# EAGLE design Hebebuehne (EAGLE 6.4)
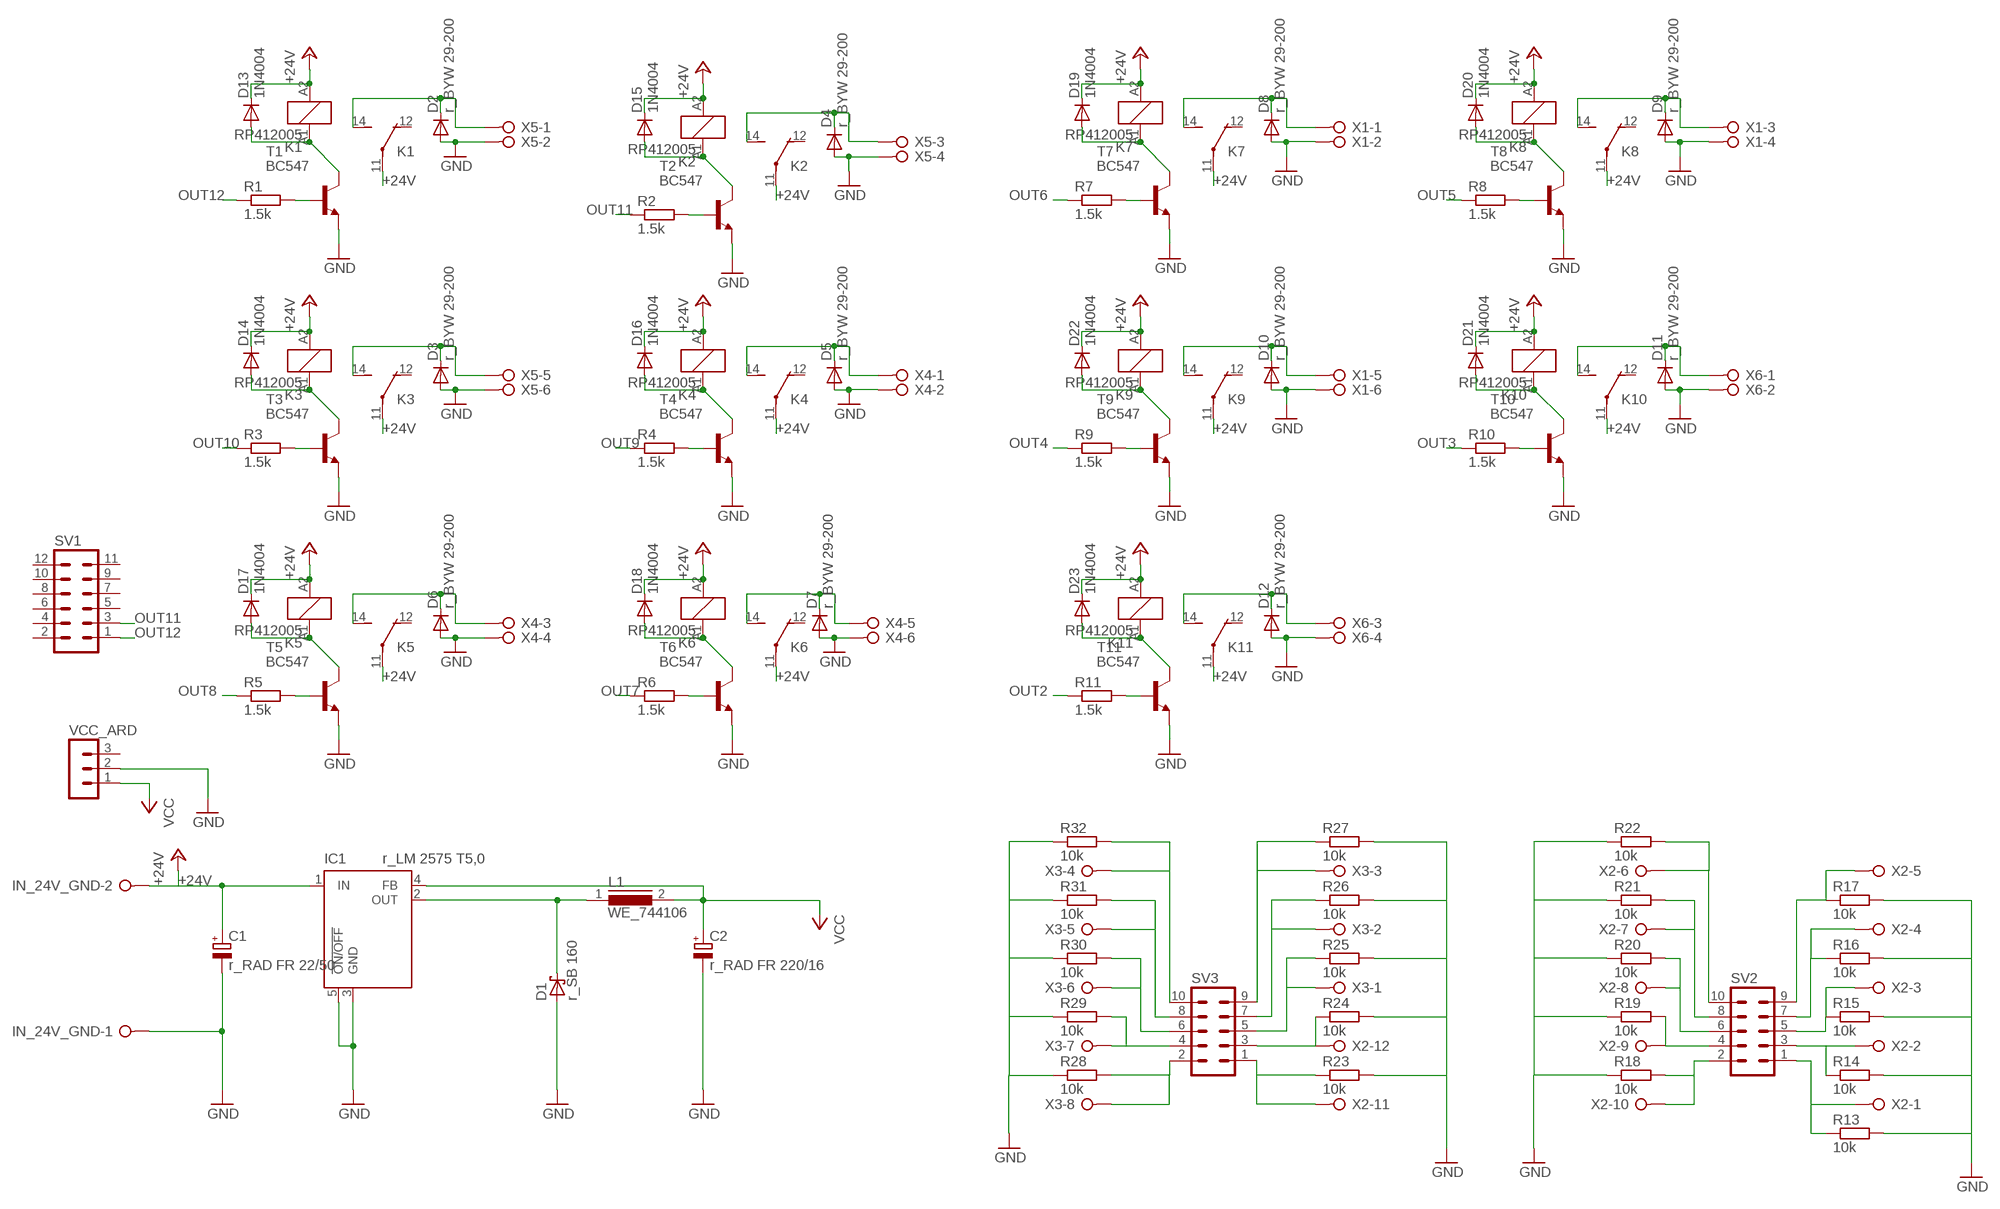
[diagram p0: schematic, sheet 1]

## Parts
C1  r_RAD FR 22/50  CPOL-EUE2.5-6  [E2,5-6]
C2  r_RAD FR 220/16  CPOL-EUE2.5-6  [E2,5-6]
D1  r_SB 160  BAT49  [DO41-10]
D2  r_BYW 29-200  MUR810  [TO220ACS]
D3  r_BYW 29-200  MUR810  [TO220ACS]
D4  r_BYW 29-200  MUR810  [TO220ACS]
D5  r_BYW 29-200  MUR810  [TO220ACS]
D6  r_BYW 29-200  MUR810  [TO220ACS]
D7  r_BYW 29-200  MUR810  [TO220ACS]
D8  r_BYW 29-200  MUR810  [TO220ACS]
D9  r_BYW 29-200  MUR810  [TO220ACS]
D10  r_BYW 29-200  MUR810  [TO220ACS]
D11  r_BYW 29-200  MUR810  [TO220ACS]
D12  r_BYW 29-200  MUR810  [TO220ACS]
D13  1N4004  [DO41-10]
D14  1N4004  [DO41-10]
D15  1N4004  [DO41-10]
D16  1N4004  [DO41-10]
D17  1N4004  [DO41-10]
D18  1N4004  [DO41-10]
D19  1N4004  [DO41-10]
D20  1N4004  [DO41-10]
D21  1N4004  [DO41-10]
D22  1N4004  [DO41-10]
D23  1N4004  [DO41-10]
IC1  r_LM 2575 T5,0  LM2575  [CB367]
IN_24V_GND  W237-02P  [W237-132]
K1  RP412005  [RT-C/O12A3.5]
K2  RP412005  [RT-C/O12A3.5]
K3  RP412005  [RT-C/O12A3.5]
K4  RP412005  [RT-C/O12A3.5]
K5  RP412005  [RT-C/O12A3.5]
K6  RP412005  [RT-C/O12A3.5]
K7  RP412005  [RT-C/O12A3.5]
K8  RP412005  [RT-C/O12A3.5]
K9  RP412005  [RT-C/O12A3.5]
K10  RP412005  [RT-C/O12A3.5]
K11  RP412005  [RT-C/O12A3.5]
L1  WE_744106  R1305D11  [11-13]
R1  1.5k  R-EU_0204/7  [0204/7]
R2  1.5k  R-EU_0204/7  [0204/7]
R3  1.5k  R-EU_0204/7  [0204/7]
R4  1.5k  R-EU_0204/7  [0204/7]
R5  1.5k  R-EU_0204/7  [0204/7]
R6  1.5k  R-EU_0204/7  [0204/7]
R7  1.5k  R-EU_0204/7  [0204/7]
R8  1.5k  R-EU_0204/7  [0204/7]
R9  1.5k  R-EU_0204/7  [0204/7]
R10  1.5k  R-EU_0204/7  [0204/7]
R11  1.5k  R-EU_0204/7  [0204/7]
R13  10k  R-EU_0207/10  [0207/10]
R14  10k  R-EU_0207/10  [0207/10]
R15  10k  R-EU_0207/10  [0207/10]
R16  10k  R-EU_0207/10  [0207/10]
R17  10k  R-EU_0207/10  [0207/10]
R18  10k  R-EU_0207/10  [0207/10]
R19  10k  R-EU_0207/10  [0207/10]
R20  10k  R-EU_0207/10  [0207/10]
R21  10k  R-EU_0207/10  [0207/10]
R22  10k  R-EU_0207/10  [0207/10]
R23  10k  R-EU_0207/10  [0207/10]
R24  10k  R-EU_0207/10  [0207/10]
R25  10k  R-EU_0207/10  [0207/10]
R26  10k  R-EU_0207/10  [0207/10]
R27  10k  R-EU_0207/10  [0207/10]
R28  10k  R-EU_0207/10  [0207/10]
R29  10k  R-EU_0207/10  [0207/10]
R30  10k  R-EU_0207/10  [0207/10]
R31  10k  R-EU_0207/10  [0207/10]
R32  10k  R-EU_0207/10  [0207/10]
SV1  MA06-2  [MA06-2]
SV2  MA05-2  [MA05-2]
SV3  MA05-2  [MA05-2]
T1  BC547  [TO92]
T2  BC547  [TO92]
T3  BC547  [TO92]
T4  BC547  [TO92]
T5  BC547  [TO92]
T6  BC547  [TO92]
T7  BC547  [TO92]
T8  BC547  [TO92]
T9  BC547  [TO92]
T10  BC547  [TO92]
T11  BC547  [TO92]
VCC_ARD  MA03-1  [MA03-1]
X1  W237-06P  [W237-6P]
X2  W237-12P  [W237-12P]
X3  W237-08P  [W237-8P]
X4  W237-06P  [W237-6P]
X5  W237-06P  [W237-6P]
X6  W237-04P  [W237-4P]

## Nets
+24V: C1.+ D13.C D14.C D15.C D16.C D17.C D18.C D19.C D20.C D21.C D22.C D23.C IC1.1(IN) IN_24V_GND.2 K1.11(2:P) K1.A2 K2.11(2:P) K2.A2 K3.11(2:P) K3.A2 K4.11(2:P) K4.A2 K5.11(2:P) K5.A2 K6.11(2:P) K6.A2 K7.11(2:P) K7.A2 K8.11(2:P) K8.A2 K9.11(2:P) K9.A2 K10.11(2:P) K10.A2 K11.11(2:P) K11.A2
GND: C1.- C2.- D1.A D2.A D3.A D4.A D5.A D6.A D7.A D8.A D9.A D10.A D11.A D12.A IC1.3(GND) IC1.5(!ON/OFF) IN_24V_GND.1 R13.2 R14.2 R15.2 R16.2 R17.2 R18.1 R19.1 R20.1 R21.1 R22.1 R23.2 R24.2 R25.2 R26.2 R27.2 R28.1 R29.1 R30.1 R31.1 R32.1 T1.1(E) T2.1(E) T3.1(E) T4.1(E) T5.1(E) T6.1(E) T7.1(E) T8.1(E) T9.1(E) T10.1(E) T11.1(E) VCC_ARD.2 X1.2 X1.4 X1.6 X4.2 X4.4 X4.6 X5.2 X5.4 X5.6 X6.2 X6.4
N$1: D5.C K4.14(2:S) X4.1
N$2: D2.C K1.14(2:S) X5.1
N$3: D1.C IC1.2(OUT) L1.1
N$4: D4.C K2.14(2:S) X5.3
N$5: D3.C K3.14(2:S) X5.5
N$6: R1.2 T1.2(B)
N$7: D13.A K1.A1 T1.3(C)
N$8: R2.2 T2.2(B)
N$9: D6.C K5.14(2:S) X4.3
N$10: D7.C K6.14(2:S) X4.5
N$11: D8.C K7.14(2:S) X1.1
N$12: D15.A K2.A1 T2.3(C)
N$13: R3.2 T3.2(B)
N$14: R9.2 T9.2(B)
N$15: D9.C K8.14(2:S) X1.3
N$16: D22.A K9.A1 T9.3(C)
N$17: D14.A K3.A1 T3.3(C)
N$18: R4.2 T4.2(B)
N$19: R10.2 T10.2(B)
N$20: D21.A K10.A1 T10.3(C)
N$21: D10.C K9.14(2:S) X1.5
N$22: D16.A K4.A1 T4.3(C)
N$23: R5.2 T5.2(B)
N$24: D11.C K10.14(2:S) X6.1
N$25: R11.2 T11.2(B)
N$26: D23.A K11.A1 T11.3(C)
N$27: D17.A K5.A1 T5.3(C)
N$28: R6.2 T6.2(B)
N$31: D12.C K11.14(2:S) X6.3
N$32: D18.A K6.A1 T6.3(C)
N$33: R7.2 T7.2(B)
N$35: R28.2 SV3.2 X3.8
N$36: R29.2 SV3.4 X3.7
N$37: D19.A K7.A1 T7.3(C)
N$38: R8.2 T8.2(B)
N$39: R22.2 SV2.10 X2.6
N$40: R32.2 SV3.10 X3.4
N$41: R31.2 SV3.8 X3.5
N$42: D20.A K8.A1 T8.3(C)
N$43: R21.2 SV2.8 X2.7
N$44: R20.2 SV2.6 X2.8
N$45: R15.1 SV2.5 X2.3
N$46: R17.1 SV2.9 X2.5
N$47: R16.1 SV2.7 X2.4
N$48: R14.1 SV2.3 X2.2
N$49: R13.1 SV2.1 X2.1
N$50: R30.2 SV3.6 X3.6
N$51: R19.2 SV2.4 X2.9
N$52: R18.2 SV2.2 X2.10
N$53: R23.1 SV3.1 X2.11
N$54: R24.1 SV3.3 X2.12
N$55: R27.1 SV3.9 X3.3
N$56: R26.1 SV3.7 X3.2
N$57: R25.1 SV3.5 X3.1
OUT2: R11.1
OUT3: R10.1
OUT4: R9.1
OUT5: R8.1
OUT6: R7.1
OUT7: R6.1
OUT8: R5.1
OUT9: R4.1
OUT10: R3.1
OUT11: R2.1 SV1.3
OUT12: R1.1 SV1.1
VCC: C2.+ IC1.4(FB) L1.2 VCC_ARD.1
Unconnected: K1.12(2:O) K2.12(2:O) K3.12(2:O) K4.12(2:O) K5.12(2:O) K6.12(2:O) K7.12(2:O) K8.12(2:O) K9.12(2:O) K10.12(2:O) K11.12(2:O) SV1.2 SV1.4 SV1.5 SV1.6 SV1.7 SV1.8 SV1.9 SV1.10 SV1.11 SV1.12 VCC_ARD.3

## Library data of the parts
C1 C2 = resistor:CPOL-EU: POLARIZED CAPACITOR, European symbol
D1 = diode:BAT49: DIODE
D2-D12 = diode:MUR810: DIODE
D13-D23 = diode:1N4004: DIODE
IC1 = eigene:LM2575
IN_24V_GND = con-wago-508:W237-02P: WAGO SREW CLAMP; OC_FARNELL: unknown; OC_NEWARK: unknown
K1-K11 = relay:RP?12*: Power PCB Relay RP II/1 SCHRACK 1 pole 8 / 12 A Source: http://www.schrack.com/.. 5834.pdf; MF: TYCO ELECTRONICS; MPN: 1393231-8; OC_FARNELL: unknown; OC_NEWARK: 11H3247
L1 = inductor-nkl:R1305D: Speicherdrossel (bis typ. 250kHz); OC_FARNELL: unknown; OC_NEWARK: unknown
R1-R11 R13-R32 = resistor:R-EU_: RESISTOR, European symbol
SV1 = con-lstb:MA06-2: PIN HEADER; OC_FARNELL: unknown; OC_NEWARK: unknown
SV2 SV3 = con-lstb:MA05-2: PIN HEADER; OC_FARNELL: unknown; OC_NEWARK: unknown
T1-T11 = transistor:BC547: NPN TRANSISTOR
VCC_ARD = con-lstb:MA03-1: PIN HEADER; OC_FARNELL: unknown; OC_NEWARK: unknown
X1 X4 X5 = con-wago-508:W237-06P: WAGO SREW CLAMP; OC_FARNELL: unknown; OC_NEWARK: unknown
X2 = con-wago-508:W237-12P: WAGO SREW CLAMP; OC_FARNELL: unknown; OC_NEWARK: unknown
X3 = con-wago-508:W237-08P: WAGO SREW CLAMP; OC_FARNELL: unknown; OC_NEWARK: unknown
X6 = con-wago-508:W237-04P: WAGO SREW CLAMP; OC_FARNELL: unknown; OC_NEWARK: unknown

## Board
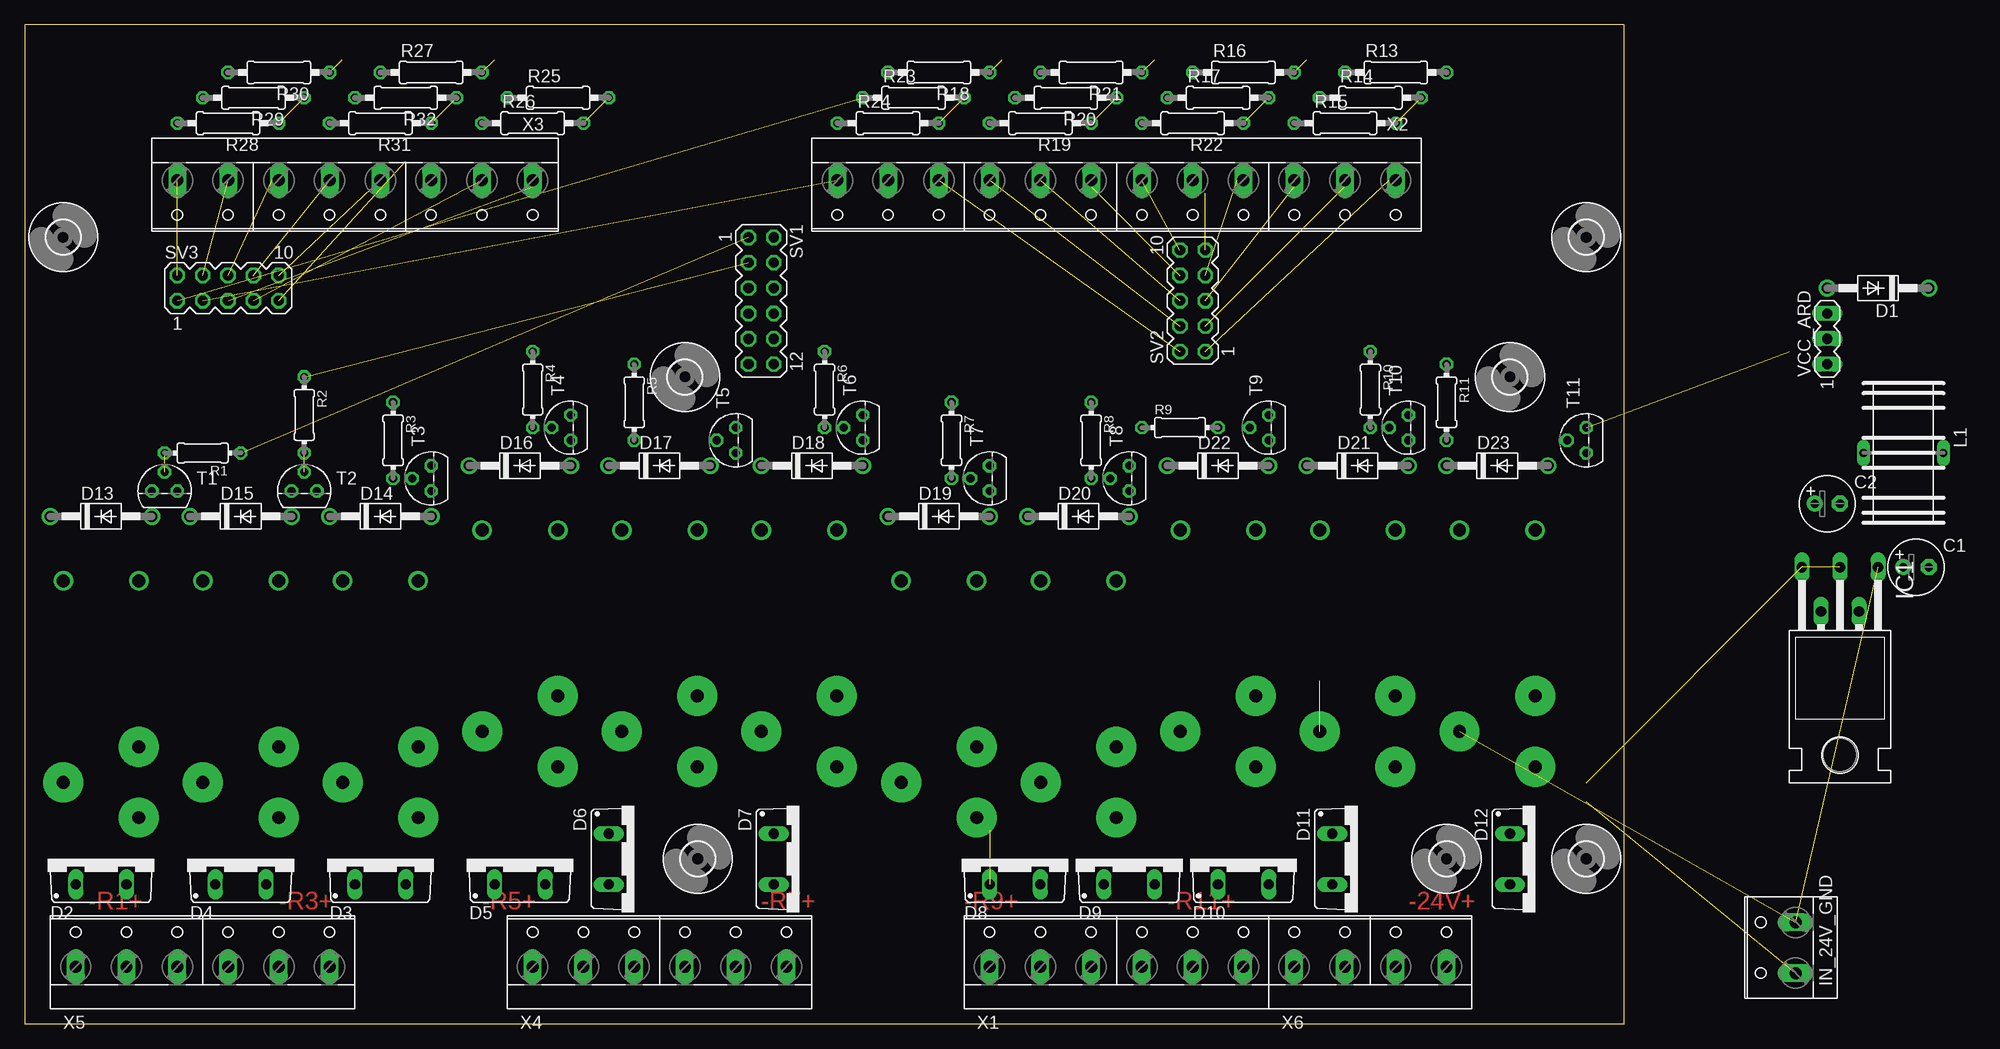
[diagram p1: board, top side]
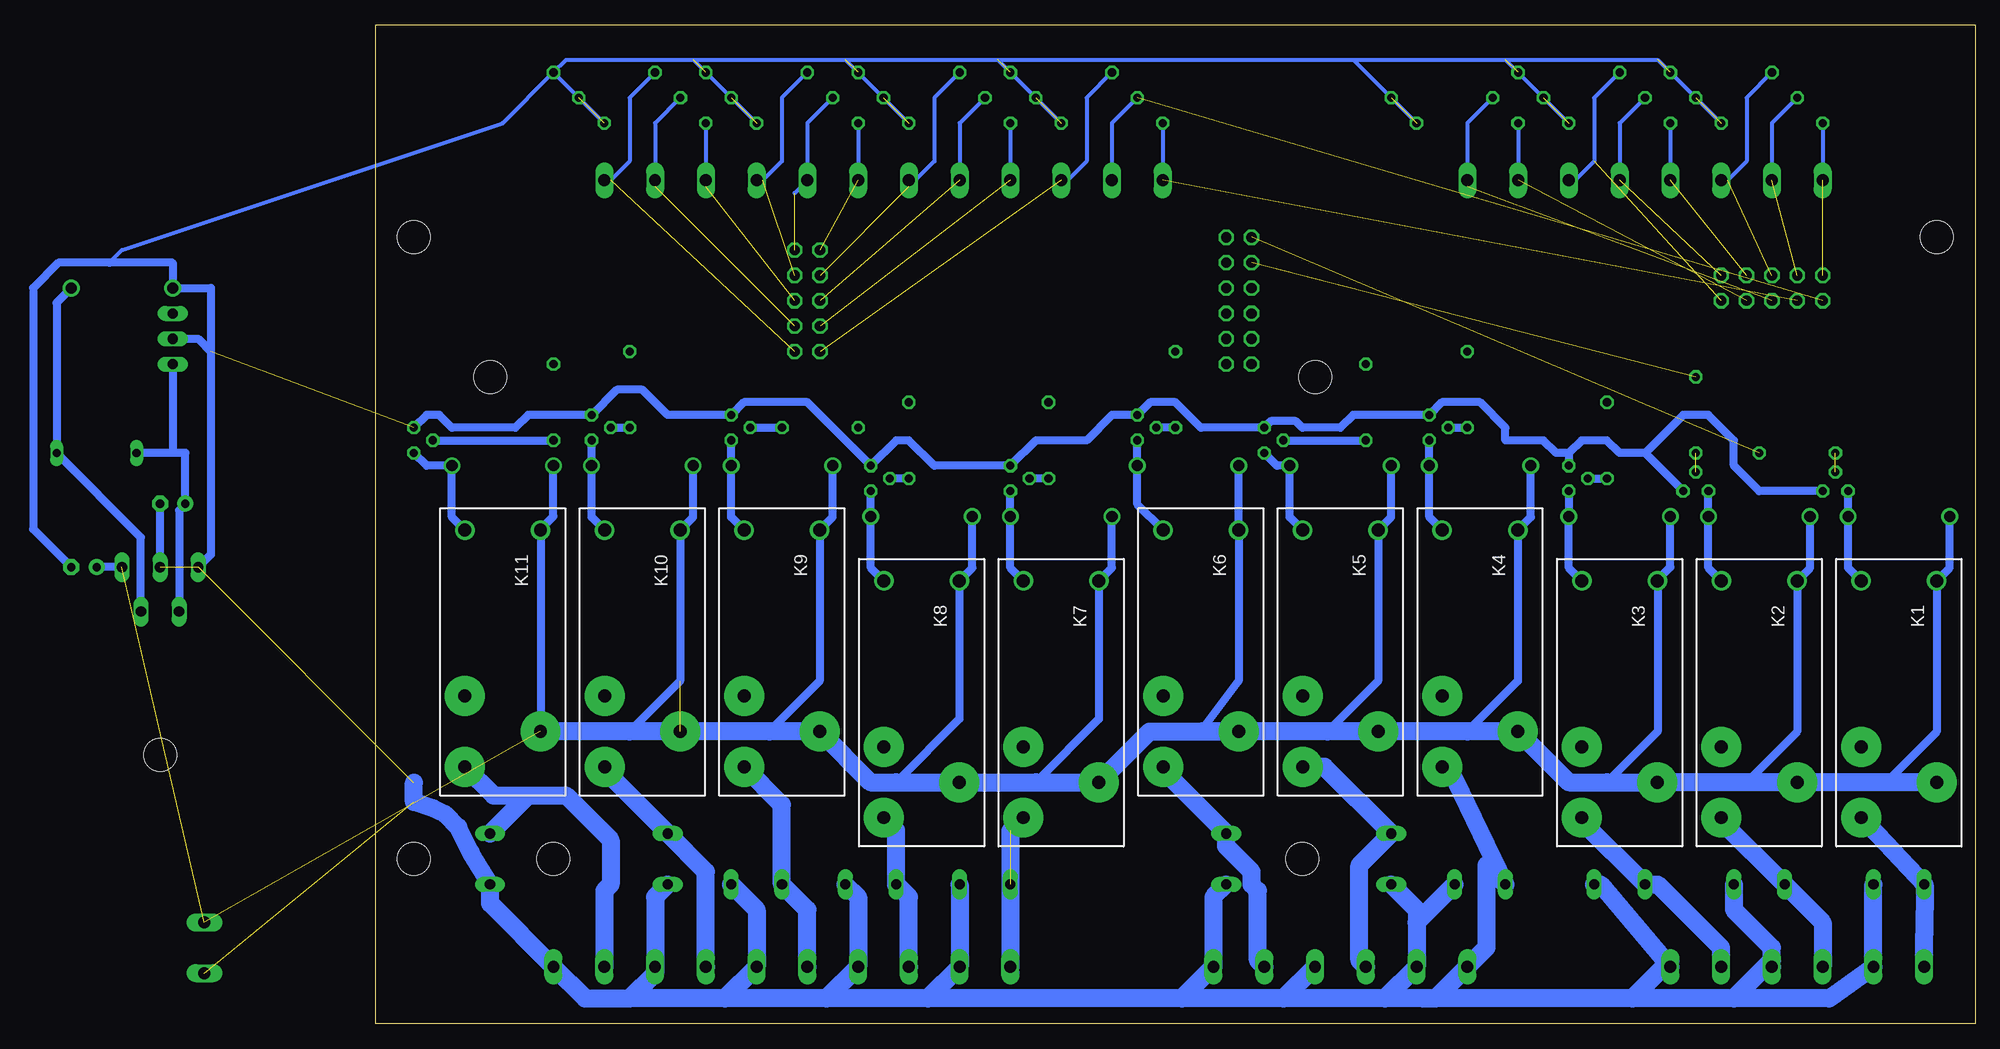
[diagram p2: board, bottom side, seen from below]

Size 160 x 100 mm. Coordinates in mm from the lower left corner, seen from the top.
Outline: 0,0 160,0 160,100 0,100 0,0
Copper layers (1*16): Top 0.035mm / dielectric 1.5mm / Bottom 0.035mm
Design rules "default": minimum track width 10mil, minimum drill 24mil, track to track 8mil, track to pad 8mil, pad to pad 8mil, via to via 8mil, smd to smd 8mil, copper to edge 40mil, drill to drill 8mil, minimum pad ring 10mil, minimum via ring 8mil, stop-mask expansion 4mil, vias tented up to drill 0mil, thermal gap 10mil

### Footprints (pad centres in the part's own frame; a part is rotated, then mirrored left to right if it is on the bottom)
E2,5-6 = drill 0.813 pad 1.6: + -1.27,0 | drill 0.813 pad 1.6 octagon: - 1.27,0
DO41-10 = drill 1.118: A 5.08,0; C -5.08,0
TO220ACS = drill 1.016 long: A 2.54,-2.54; C -2.54,-2.54
CB367 = drill 1.016 long: 1 -3.81,-11.43; 2 -1.905,-6.985; 3 0,-11.43; 4 1.905,-6.985; 5 3.81,-11.43 | hole 3.302: 0,7.366
W237-132 = drill 1.194 long: 1 -2.54,-0.635; 2 2.54,-0.635
RT-C/O12A3.5 = drill 1.3 pad 4: 11 7.56,3.78; 12 4.02,-3.78; 14 11.1,-3.78 | drill 1.3: A1 -12.6,-3.78; A2 -12.6,3.78
11-13 = drill 0.813 long: 1 -4,0; 2 4,0
0204/7 = drill 0.813 octagon: 1 -3.81,0; 2 3.81,0
0207/10 = drill 0.813 octagon: 1 -5.08,0; 2 5.08,0
MA06-2 = drill 1.016 octagon: 1 -6.35,-1.27; 2 -6.35,1.27; 3 -3.81,-1.27; 4 -3.81,1.27; 5 -1.27,-1.27; 6 -1.27,1.27; 7 1.27,-1.27; 8 1.27,1.27; 9 3.81,-1.27; 10 3.81,1.27; 11 6.35,-1.27; 12 6.35,1.27
MA05-2 = drill 1.016 octagon: 1 -5.08,-1.27; 2 -5.08,1.27; 3 -2.54,-1.27; 4 -2.54,1.27; 5 0,-1.27; 6 0,1.27; 7 2.54,-1.27; 8 2.54,1.27; 9 5.08,-1.27; 10 5.08,1.27
TO92 = drill 0.813 octagon: 1 1.27,0; 2 0,1.905; 3 -1.27,0
3,3 = hole 3.3: 0,0
MA03-1 = drill 1.016 long: 1 -2.54,0; 2 0,0; 3 2.54,0
W237-6P = drill 1.194 long: 1 -12.7,-0.635; 2 -7.62,-0.635; 3 -2.54,-0.635; 4 2.54,-0.635; 5 7.62,-0.635; 6 12.7,-0.635
W237-12P = drill 1.194 long: 1 -27.94,-0.635; 2 -22.86,-0.635; 3 -17.78,-0.635; 4 -12.7,-0.635; 5 -7.62,-0.635; 6 -2.54,-0.635; 7 2.54,-0.635; 8 7.62,-0.635; 9 12.7,-0.635; 10 17.78,-0.635; 11 22.86,-0.635; 12 27.94,-0.635
W237-8P = drill 1.194 long: 1 -17.78,-0.635; 2 -12.7,-0.635; 3 -7.62,-0.635; 4 -2.54,-0.635; 5 2.54,-0.635; 6 7.62,-0.635; 7 12.7,-0.635; 8 17.78,-0.635
W237-4P = drill 1.194 long: 1 -7.62,-0.635; 2 -2.54,-0.635; 3 2.54,-0.635; 4 7.62,-0.635

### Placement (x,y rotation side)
C1  189.23,45.72 0 top  (outside the outline)
C2  180.34,52.07 0 top  (outside the outline)
D1  185.42,73.66 180 top  (outside the outline)
D2  7.62,16.51 0 top
D3  35.56,16.51 0 top
D4  21.59,16.51 0 top
D5  49.53,16.51 0 top
D6  60.96,16.51 270 top
D7  77.47,16.51 270 top
D8  99.06,16.51 0 top
D9  110.49,16.51 0 top
D10  121.92,16.51 0 top
D11  133.35,16.51 270 top
D12  151.13,16.51 270 top
D13  7.62,50.8 0 top
D14  35.56,50.8 0 top
D15  21.59,50.8 0 top
D16  49.53,55.88 0 top
D17  63.5,55.88 0 top
D18  78.74,55.88 0 top
D19  91.44,50.8 0 top
D20  105.41,50.8 0 top
D21  133.35,55.88 0 top
D22  119.38,55.88 0 top
D23  147.32,55.88 0 top
IC1  181.61,34.29 180 top  (outside the outline)
IN_24V_GND  not placed on the board
K1  7.62,31.75 270 bottom
K2  21.59,31.75 270 bottom
K3  35.56,31.75 270 bottom
K4  49.53,36.83 270 bottom
K5  63.5,36.83 270 bottom
K6  77.47,36.83 270 bottom
K7  91.44,31.75 270 bottom
K8  105.41,31.75 270 bottom
K9  119.38,36.83 270 bottom
K10  133.35,36.83 270 bottom
K11  147.32,36.83 270 bottom
L1  187.96,57.15 180 top  (outside the outline)
R1  17.78,57.15 180 top
R2  27.94,60.96 270 top
R3  36.83,58.42 270 top
R4  50.8,63.5 270 top
R5  60.96,62.23 270 top
R6  80.01,63.5 270 top
R7  92.71,58.42 270 top
R8  106.68,58.42 270 top
R9  115.57,59.69 0 top
R10  134.62,63.5 270 top
R11  142.24,62.23 270 top
R13  137.16,95.25 0 top
R14  134.62,92.71 0 top
R15  132.08,90.17 0 top
R16  121.92,95.25 0 top
R17  119.38,92.71 0 top
R18  91.44,95.25 180 top
R19  101.6,90.17 180 top
R20  104.14,92.71 180 top
R21  106.68,95.25 180 top
R22  116.84,90.17 180 top
R23  88.9,92.71 0 top
R24  86.36,90.17 0 top
R25  53.34,92.71 0 top
R26  50.8,90.17 0 top
R27  40.64,95.25 0 top
R28  20.32,90.17 180 top
R29  22.86,92.71 180 top
R30  25.4,95.25 180 top
R31  35.56,90.17 180 top
R32  38.1,92.71 180 top
SV1  73.66,72.39 270 top
SV2  116.84,72.39 90 top
SV3  20.32,73.66 0 top
T1  13.97,53.34 0 top
T2  27.94,53.34 0 top
T3  40.64,54.61 90 top
T4  54.61,59.69 90 top
T5  71.12,58.42 90 top
T6  83.82,59.69 90 top
T7  96.52,54.61 90 top
T8  110.49,54.61 90 top
T9  124.46,59.69 90 top
T10  138.43,59.69 90 top
T11  156.21,58.42 90 top
U$1  [3,3]  67.31,16.51 0 top
U$2  [3,3]  66.04,64.77 0 top
U$3  [3,3]  156.21,16.51 0 top
U$4  [3,3]  148.59,64.77 0 top
U$5  [3,3]  not placed on the board
U$6  [3,3]  3.81,78.74 0 top
U$7  [3,3]  142.24,16.51 0 top
U$8  [3,3]  156.21,78.74 0 top
VCC_ARD  180.34,68.58 90 top  (outside the outline)
X1  109.22,6.35 0 top
X2  109.22,83.82 180 top
X3  33.02,83.82 180 top
X4  63.5,6.35 0 top
X5  17.78,6.35 0 top
X6  134.62,6.35 0 top

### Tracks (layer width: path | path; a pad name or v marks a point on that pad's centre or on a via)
+24V  (3 unrouted)
  Bottom 0.813: IC1.1 C1.+ | 50.8,29.27 45.75,34.32 K4.A2 44.45,50.73 D16.C | 64.77,29.27 59.72,34.32 K5.A2 58.42,50.73 D17.C | 77.47,29.27 73.69,34.32 K6.A2 73.66,49.46 D18.C | 120.65,29.27 115.6,34.32 K9.A2 114.3,50.73 D22.C | 134.62,29.27 129.57,34.32 K10.A2 128.27,50.73 D21.C | K11.A2 143.54,49.5 143.51,49.53 | 143.51,49.53 143.51,29.3 K11.11 | 93.98,24.19 87.66,30.51 K7.A2 86.36,45.65 D19.C | 107.95,24.19 101.63,30.51 K8.A2 100.33,45.65 D20.C | 8.89,24.19 3.84,29.24 K1.A2 2.54,45.65 D13.C | 22.86,24.19 17.81,29.24 K2.A2 16.51,45.65 D15.C | K3.A2 31.78,44.42 31.75,44.45 | 31.75,44.45 31.75,29.27 36.83,24.19 | 31.75,44.45 30.48,45.72 D14.C | 143.51,49.53 142.24,50.8 D23.C
  Bottom 1.778: K6.11 64.77,29.27 K5.11 50.8,29.27 K4.11 40.67,24.19 36.83,24.19 K3.11 22.86,24.19 K2.11 8.89,24.19 K1.11 | K6.11 77.47,29.27 | K8.11 101.63,24.22 | K11.11 134.62,29.27 120.65,29.27 K9.11 110.52,24.19 107.95,24.19 K8.11 | K8.11 93.98,24.19 K7.11 82.58,29.27 K6.11
GND  (16 unrouted)
  Bottom 0.406: 186.69,76.2 185.42,77.47 147.32,90.17 R13.2 | R13.2 140.97,96.52 128.27,96.52 | 128.27,96.52 113.03,96.52 | 113.03,96.52 97.79,96.52 | 97.79,96.52 62.23,96.52 | 62.23,96.52 46.99,96.52 | 46.99,96.52 31.75,96.52 R28.1 | R31.1 46.99,96.52 | R26.2 62.23,96.52 | R24.2 97.79,96.52 | R19.1 113.03,96.52 | R22.1 128.27,96.52 | R15.2 R13.2
  Bottom 0.813: 181.61,46.99 IC1.3 C2.- | 176.53,67.31 176.53,73.66 D1.A 180.34,76.2 186.69,76.2 191.77,76.2 194.31,73.66 194.31,49.53 C1.- | 176.53,67.31 176.53,46.99 IC1.5 | VCC_ARD.2 177.8,68.58 176.53,67.31 | T1.1 21.59,53.34 24.13,55.88 24.13,58.42 26.67,60.96 29.21,60.96 33.02,57.15 | 33.02,57.15 35.56,57.15 36.83,58.42 39.37,58.42 40.64,57.15 | 40.64,57.15 T3.1 | T2.1 33.02,57.15 | 40.64,57.15 41.91,57.15 43.18,58.42 46.99,58.42 46.99,59.69 49.53,62.23 53.34,62.23 T4.1 62.23,60.96 63.5,59.69 67.31,59.69 67.94,60.33 70.48,60.33 T5.1 77.47,59.69 80.01,62.23 82.55,62.23 T6.1 86.36,60.96 88.9,58.42 93.98,58.42 T7.1 104.14,55.88 106.68,58.42 107.95,58.42 T8.1 116.84,62.23 123.19,62.23 T9.1 130.81,60.96 133.35,63.5 135.89,63.5 T10.1 144.78,60.96 146.05,59.69 152.4,59.69 153.67,60.96 154.94,60.96 T11.1
  Bottom 1.778: D4.A 24.13,11.43 20.32,7.62 X5.4 20.32,6.35 24.13,2.54 | D2.A X5.2 14.61,2.54 24.13,2.54 | 24.13,2.54 34.29,2.54 | 34.29,2.54 59.05,2.54 | 59.05,2.54 69.22,2.54 | 69.22,2.54 79.38,2.54 | 79.38,2.54 104.78,2.54 | 104.78,2.54 114.94,2.54 | 114.94,2.54 125.09,2.54 | 34.29,2.54 30.48,6.35 X5.6 37.47,13.97 D3.A | D5.A 55.88,10.16 X4.2 | D6.A 55.88,11.43 X4.2 | X4.2 59.05,2.54 | X4.4 69.22,2.54 | X4.6 79.38,2.54 | D7.A 76.2,12.7 X4.6 | 76.2,10.16 X4.6 | 104.78,2.54 X1.2 D8.A | 114.94,2.54 X1.4 111.76,12.7 D9.A | 125.09,2.54 X1.6 121.92,11.43 D10.A | 125.09,2.54 134.62,2.54 | D11.A 132.08,12.7 X6.2 132.08,5.08 134.62,2.54 | 134.62,2.54 139.06,2.54 X6.4 148.59,12.06 D12.A 150.5,17.14 151.76,19.68 153.03,20.95 154.31,21.59 156.21,22.23 156.21,24.13
N$1
  Bottom 1.778: K4.14 52.07,24.49 D5.C 48.9,15.88 48.9,7.62 X4.1 53.98,2.54 55.24,2.54
N$2
  Bottom 1.778: K1.14 5.05,13.94 | 5.05,13.94 5.08,8.89 X5.1 | 5.05,13.94 D2.C
N$3
  Bottom 0.813: IC1.2 183.51,48.7 L1.1 191.96,72.2 D1.C
N$4
  Bottom 1.778: X5.3 15.24,10.16 D4.C 25.37,20.29 K2.14
N$5
  Bottom 1.778: X5.5 25.4,7.62 31.75,13.97 D3.C 39.34,20.29 K3.14
N$6  (1 unrouted)
N$7
  Bottom 0.813: K1.A1 12.7,45.65 D13.A T1.3
N$8  (1 unrouted)
N$9
  Bottom 1.778: X4.3 61.59,6.35 61.59,15.88 D6.C 65.1,25.73 K5.14
N$10
  Bottom 1.778: X4.5 71.75,6.35 71.75,13.34 72.39,13.97 72.39,15.24 74.93,17.78 D7.C 81.25,25.37 K6.14
N$11  (1 unrouted)
  Bottom 1.778: K7.14 96.52,19.35 X1.1 96.52,5.08
N$12
  Bottom 0.813: K2.A1 26.67,45.65 D15.A T2.3
N$13
  Bottom 0.813: T3.2 R3.2
N$14
  Bottom 0.813: T9.2 R9.2
N$15
  Bottom 1.778: X1.3 106.68,12.7 D9.C 107.95,19.41 K8.14
N$16
  Bottom 0.813: K9.A1 124.46,50.73 D22.A T9.3
N$17
  Bottom 0.813: K3.A1 40.64,45.65 D14.A T3.3
N$18
  Bottom 0.813: T4.2 R4.2
N$19
  Bottom 0.813: T10.2 R10.2
N$20
  Bottom 0.813: K10.A1 138.43,50.73 D21.A T10.3
N$21
  Bottom 1.778: X1.5 116.84,11.43 D10.C 119.38,21.95 K9.14
N$22
  Bottom 0.813: K4.A1 54.61,50.73 D16.A T4.3
N$23
  Bottom 0.813: T5.2 R5.2
N$24
  Bottom 1.778: X6.1 127,15.24 D11.C 137.13,25.37 K10.14
N$25
  Bottom 0.813: T11.2 R11.2
N$26
  Bottom 0.813: K11.A1 152.4,50.73 D23.A 154.94,55.88 T11.3
N$27
  Bottom 0.813: K5.A1 68.58,50.73 D17.A 69.85,55.88 T5.3
N$28
  Bottom 0.813: R6.2 T6.2
N$31
  Bottom 1.778: D12.C 144.78,22.86 | 144.78,22.86 143.51,22.86 140.97,22.86 136.53,18.41 136.53,13.97 137.16,13.34 X6.3 | K11.14 148.23,22.86 144.78,22.86
N$32
  Bottom 0.813: K6.A1 83.82,52 D18.A T6.3
N$33
  Bottom 0.813: R7.2 T7.2
N$35  (1 unrouted)
  Bottom 0.406: R28.2 X3.8
N$36  (1 unrouted)
  Bottom 0.406: R29.2 20.32,90.17 X3.7
N$37
  Bottom 0.813: K7.A1 96.52,45.65 D19.A T7.3
N$38
  Bottom 0.813: R8.2 T8.2
N$39  (1 unrouted)
  Bottom 0.406: R22.2 X2.6
N$40  (1 unrouted)
  Bottom 0.406: R32.2 35.56,90.17 X3.4
N$41  (1 unrouted)
  Bottom 0.406: R31.2 X3.5
N$42
  Bottom 0.813: K8.A1 110.49,45.65 D20.A T8.3
N$43  (1 unrouted)
  Bottom 0.406: 106.68,83.82 X2.7 106.05,84.45 104.14,86.36 104.14,92.71 R21.2
N$44  (1 unrouted)
  Bottom 0.406: R20.2 101.6,90.17 X2.8
N$45  (1 unrouted)
  Bottom 0.406: 127,83.82 X2.3 R15.1
N$46  (1 unrouted)
  Bottom 0.406: 118.11,83.19 X2.5 116.84,90.17 R17.1
N$47  (1 unrouted)
  Bottom 0.406: R16.1 119.38,92.71 119.38,86.36 121.28,84.45 X2.4
N$48  (1 unrouted)
  Bottom 0.406: 132.08,83.82 X2.2 132.08,90.17 R14.1
N$49  (1 unrouted)
  Bottom 0.406: R13.1 134.62,92.71 134.62,86.36 136.53,84.45 X2.1
N$50  (1 unrouted)
  Bottom 0.406: R30.2 22.86,92.71 22.86,86.36 24.77,84.45 X3.6
N$51  (1 unrouted)
  Bottom 0.406: R19.2 X2.9
N$52  (1 unrouted)
  Bottom 0.406: R18.2 88.9,92.71 88.9,86.36 90.81,84.45 X2.10
N$53  (1 unrouted)
  Bottom 0.406: R23.1 86.36,90.17 X2.11
N$54  (1 unrouted)
  Bottom 0.406: R24.1 X2.12
N$55  (1 unrouted)
  Bottom 0.406: 40.64,83.82 X3.3 40.01,84.45 38.1,86.36 38.1,92.71 R27.1
N$56  (1 unrouted)
  Bottom 0.406: R26.1 X3.2
N$57  (1 unrouted)
  Bottom 0.406: 50.8,83.82 X3.1 50.8,90.17 R25.1
OUT11  (1 unrouted)
OUT12  (1 unrouted)
VCC
  Bottom 0.813: IC1.4 179.71,51.44 C2.+ 179.07,57.15 180.34,57.15 | 180.34,57.15 L1.2 | VCC_ARD.1 180.34,57.15

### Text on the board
Top: -R1+ | -R3+ | -R5+ | -R7+ | -R9+ | -R11+ | -24V+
